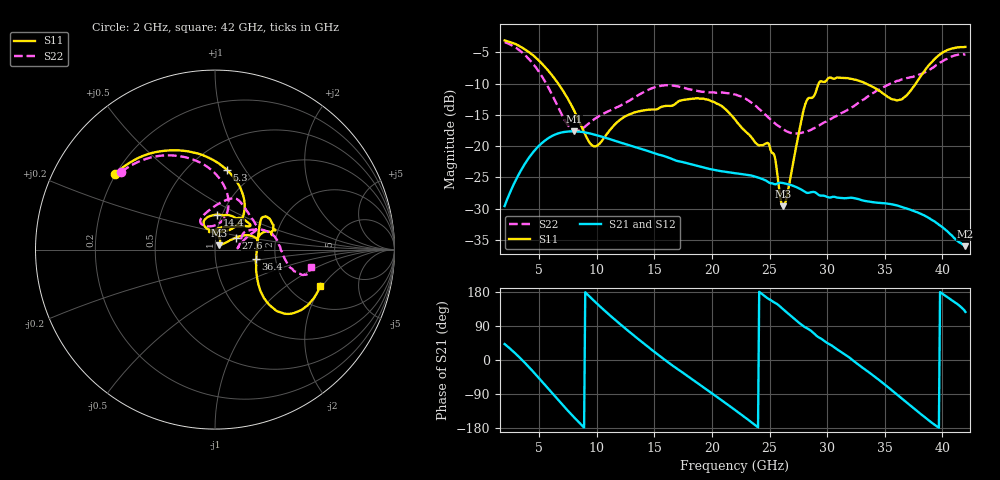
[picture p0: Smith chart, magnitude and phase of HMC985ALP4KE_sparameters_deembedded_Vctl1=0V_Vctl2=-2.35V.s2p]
!s2p File: Measurements: S11, S21, S12, S22
# GHz S dB R 50.0
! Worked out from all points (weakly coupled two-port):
!   401 points, 2 GHz to 42 GHz, reference 50 ohm
!   highest |S21| = -17.64 dB at 8 GHz (marker M1); lowest = -36.0 dB at 42 GHz (marker M2)
!   lowest |S11| = -29.6 dB at 26.2 GHz (marker M3), VSWR 1.07, Z = 52.3 + j2.48 ohm
!   |S11| at or under -10 dB: 6.648 GHz to 29.26 GHz (22.62 GHz wide, 126 % of centre); 33.37 GHz to 37.7 GHz (4.325 GHz wide, 12.2 % of centre)
!   |S22| runs from -18.0 to -3.4 dB; largest |S21 - S12| = 0.00053
!   S11 on the Smith chart (normalised r, x): 2 GHz: 0.20, +0.32; 5.3 GHz: 0.74, +0.83; 14.4 GHz: 0.95, +0.38; 27.6 GHz: 1.25, +0.17; 36.4 GHz: 1.58, -0.18; 42 GHz: 2.90, -1.91
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2  -3.12 143.0  -29.59 42.2  -29.57 42.2  -3.37 140.2
3.5  -4.24 116.0  -23.64 0.6  -23.65 0.6  -5.01 111.7
5.3  -6.94 81.7  -19.42 -58.8  -19.44 -58.9  -9.03 81.3
8  -14.19 47.9  -17.64 -150.3  -17.62 -150.2  -17.53 93.0
8.7  -16.99 52.4  -17.73 -172.2  -17.73 -172.2  -17.28 108.5
9.9  -20.04 87.5  -18.22 152.2  -18.21 152.2  -15.57 118.2
12.2  -15.56 112.2  -19.52 90.3  -19.50 90.3  -13.39 102.1
14.4  -14.20 87.0  -20.77 35.8  -20.75 35.9  -11.06 78.3
15.4  -13.95 73.3  -21.38 12.4  -21.39 12.3  -10.42 71.3
19.3  -12.44 34.1  -23.43 -72.8  -23.44 -72.9  -11.33 42.7
22  -15.75 52.3  -24.33 -131.8  -24.36 -131.9  -11.75 26.0
25  -19.99 98.8  -25.89 159.6  -25.85 159.6  -15.63 17.4
26.2  -29.61 45.6  -25.92 133.3  -25.96 133.3  -17.34 8.3
27.6  -17.36 29.8  -26.80 97.2  -26.81 97.2  -17.92 3.8
28.1  -13.30 20.9  -27.35 86.1  -27.39 86.0  -17.75 5.7
28.7  -12.27 13.0  -27.33 74.4  -27.33 74.4  -17.29 10.0
31  -9.06 23.3  -28.26 25.4  -28.25 25.3  -14.96 29.3
33.3  -9.93 34.2  -28.77 -25.2  -28.76 -25.3  -12.39 27.5
35.4  -12.27 12.0  -29.23 -74.5  -29.23 -74.6  -10.12 18.5
36.4  -12.58 -13.1  -29.68 -99.6  -29.71 -99.6  -9.38 12.7
39.5  -5.82 -43.4  -32.29 -174.5  -32.31 -174.5  -7.04 -14.1
42  -4.15 -19.0  -36.00 126.8  -35.99 126.8  -5.33 -10.4
